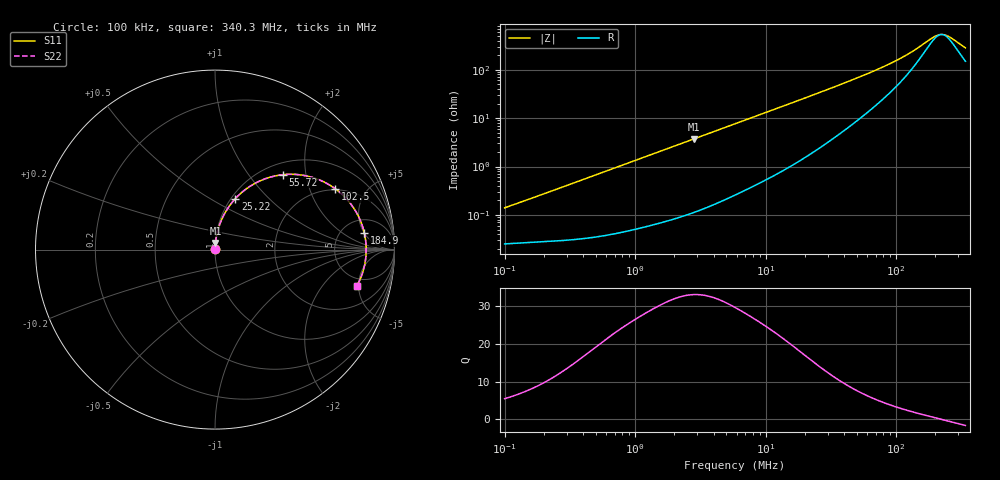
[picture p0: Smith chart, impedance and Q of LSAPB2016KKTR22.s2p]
! LSAPB2016KKTR22  S-PARAMETER MODEL  ( General Type )
! Model Generated by TAIYO YUDEN Corporation (http://www.ty-top.com)
! Version 1.0
! TAIYO YUDEN Control No. 171016NI43SB-FBB
! Copyright(c) 2017 TAIYO YUDEN CO.,LTD. All Rights Reserved.
! Product Description (link to TY-COMPAS)
! https://ds.yuden.co.jp/TYCOMPAS/or/detail?pn=LSAPB2016KKTR22M&u=M
! Products Name : Inductors
! Characteristics :
!  Inductance : 0.22 uH , SRF(min) : -Hz , DC Resistance(max) : 0.026 Ohm
!  Rated Current : Saturation :5800 mA , Temp Rise : 4000 mA (40 degC)
!  Case Size : 2.0 x 1.6 / 0.079 x 0.063 [mm/inch] , Thickness : 1 / 0.039 [mm/inch]
!  (Conditions: Temperature = 25 degC , DC Bias Current/Voltage = 0A / 0V)
! External Node Assignments :
!  1  o---GGG---o  2
! GND o---------o GND
! Frequency Range : 0.1MHz  -  340.31115MHz  [ 402 STEP ]
# MHz S RI R 50
! Freq[MHz].  S11 Real  S11 Imag  S21 Real  S21 Imag  S12 Real  S12 Imag  S22 Real  S22 Imag
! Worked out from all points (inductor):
!   401 points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, 100 kHz to 340.3 MHz, reference 50 ohm
!   read as one part in series: L = 218 nH near 104.2 kHz
!   highest Q = 33.1 at 2.806 MHz (marker M1), where L = 209 nH
!   self-resonance near 223.7 MHz
!   S11 on the Smith chart (normalised r, x): 100 kHz: 1.00, +0.00; 25.22 MHz: 1.05, +0.65; 55.72 MHz: 1.22, +1.49; 102.5 MHz: 1.95, +3.04; 184.9 MHz: 8.09, +5.05; 340.3 MHz: 3.98, -4.80
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0.1  0.000254 0.00138  0.9997 -0.00138  0.9997 -0.00138  0.000254 0.00138
0.390471  0.000349 0.00525  0.9997 -0.00525  0.9997 -0.00525  0.000349 0.00525
1.524679  0.00108 0.0202  0.9989 -0.0202  0.9989 -0.0202  0.00108 0.0202
2.805881  0.00247 0.0368  0.9975 -0.0368  0.9975 -0.0368  0.00247 0.0368
5.953437  0.00857 0.0768  0.9914 -0.0768  0.9914 -0.0768  0.00857 0.0768
8.940496  0.0176 0.1135  0.9824 -0.1135  0.9824 -0.1135  0.0176 0.1135
13.15606  0.0353 0.163  0.9647 -0.163  0.9647 -0.163  0.0353 0.163
22.77862  0.0947 0.2622  0.9053 -0.2622  0.9053 -0.2622  0.0947 0.2622
25.21598  0.1131 0.2837  0.8869 -0.2837  0.8869 -0.2837  0.1131 0.2837
37.10564  0.2144 0.3645  0.7856 -0.3645  0.7856 -0.3645  0.2144 0.3645
55.7229  0.3801 0.4175  0.6199 -0.4175  0.6199 -0.4175  0.3801 0.4175
71.11972  0.4992 0.4126  0.5008 -0.4126  0.5008 -0.4126  0.4992 0.4126
88.94399  0.6077 0.3766  0.3923 -0.3766  0.3923 -0.3766  0.6077 0.3766
102.5473  0.6708 0.3384  0.3292 -0.3384  0.3292 -0.3384  0.6708 0.3384
136.3139  0.7715 0.2332  0.2285 -0.2332  0.2285 -0.2332  0.7715 0.2332
184.9207  0.8318 0.0934  0.1682 -0.0934  0.1682 -0.0934  0.8318 0.0934
200.5877  0.8389 0.0538  0.1611 -0.0538  0.1611 -0.0538  0.8389 0.0538
213.203  0.8418 0.0237  0.1582 -0.0237  0.1582 -0.0237  0.8418 0.0237
236.0162  0.8416 -0.0264  0.1584 0.0264  0.1584 0.0264  0.8416 -0.0264
261.2704  0.8355 -0.0764  0.1645 0.0764  0.1645 0.0764  0.8355 -0.0764
326.7509  0.8011 -0.1823  0.1989 0.1823  0.1989 0.1823  0.8011 -0.1823
340.3111  0.7918 -0.2006  0.2082 0.2006  0.2082 0.2006  0.7918 -0.2006
